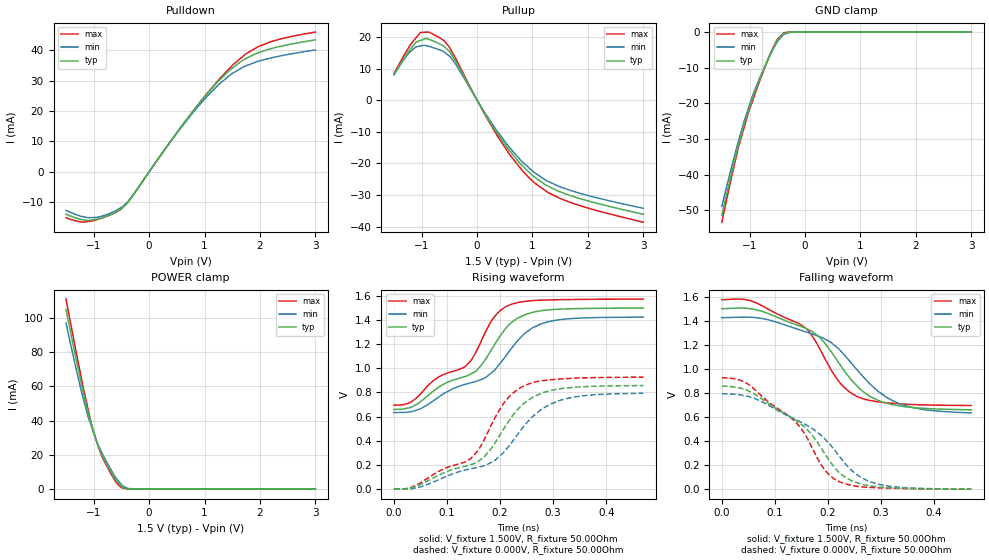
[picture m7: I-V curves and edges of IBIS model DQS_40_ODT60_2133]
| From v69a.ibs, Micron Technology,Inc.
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| MODEL DQS_40_ODT60_2133 (40 Ohm Data Strobe I/O with 60ohm ODT, 1866/2133 Mbps)
[Model]   DQS_40_ODT60_2133
Model_type   I/O
Vinl = 625.000mV
Vinh = 875.000mV
Vmeas = 750.000mV
Vref = 750.000mV
Cref = 0.0pF
Rref = 25.000Ohm
|   typ   min   max
C_comp   1.20pF   1.05pF   1.36pF
| Note: C_comp changes when the ODT circuit is enabled.
[Model Spec]
| Input threshold voltage corners
Vinl   0.6250V   0.5875V   0.6625V
Vinh   0.8750V   0.8375V   0.9125V
| Measurement voltage corners
Vmeas   0.7500V   0.7125V   0.7875V
| Timing spec test load voltage corners
Vref   0.7500V   0.7125V   0.7875V
|[Receiver Thresholds]
|Vth   =  0.750V
|Vth_min  =  0.735V
|Vth_max  =  0.765V
|Vinh_ac  =  0.125V
|Vinh_dc  =  0.100V
|Vinl_ac  = -0.125V
|Vinl_dc  = -0.100V
|Tslew_ac =  5.000ns |Not specified, so set to high value
|Threshold_sensitivity = 0.50
|Reference_supply Pullup_ref
[Receiver Thresholds]
Vcross_low   = 0.625V
Vcross_high  = 0.875V
Vdiff_ac   = 250mV
Vdiff_dc   = 200mV
Tdiffslew_ac = 10.000ns |Not specified, so set to high value
[Voltage Range]   1.5000V   1.4250V   1.5750V
[Pullup Reference]   1.5000V   1.4250V   1.5750V
| Junction Temperature (Ambient temp is 35C typ, 95C min, 0C max)
[Temperature Range]   50.0   110.0   0.0
[Add Submodel]
| Submodel Name   Mode
60ohm_ODT_2133   Non-Driving
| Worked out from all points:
|   slope of the pulldown table from 0 to 0.225 V, typ, clamps not added: 38 ohm
|   slope of the pullup table from 0 to 0.225 V, typ, clamps not added: 33.9 ohm
|   GND clamp passes 1 mA (typ) near -0.42 V on its own axis
|   POWER clamp passes 1 mA (typ) near -0.46 V on its own axis
|   falling waveform, V_fixture 1.500V, R_fixture 50.00Ohm: 20-80 % time 101ps typ, 116ps min, 91.5ps max; typ from 1.5 V to 0.659 V
|   rising waveform, V_fixture 1.500V, R_fixture 50.00Ohm: 20-80 % time 132ps typ, 147ps min, 117ps max; typ from 0.659 V to 1.5 V
|   rising waveform, V_fixture 0.000V, R_fixture 50.00Ohm: 20-80 % time 121ps typ, 135ps min, 108ps max; typ from 0 V to 0.857 V
|   falling waveform, V_fixture 0.000V, R_fixture 50.00Ohm: 20-80 % time 118ps typ, 131ps min, 107ps max; typ from 0.857 V to 0 V
[Pulldown]
|   Voltage   I(typ)   I(min)   I(max)
-1.5V     -13.96mA   -12.69mA   -15.12mA
-1.195V   -15.78mA   -14.77mA   -16.58mA
-955mV    -15.63mA   -15.03mA   -15.81mA
-495mV    -12.08mA   -11.62mA   -12.1mA
-260mV    -6.957mA   -6.872mA   -6.856mA
800mV     20.15mA    19.66mA    20.12mA
1.255V    29.89mA    28.72mA    30.25mA
1.455V    33.47mA    31.73mA    34.11mA
1.74V     37.18mA    34.8mA     38.71mA
1.975V    39.19mA    36.38mA    41.24mA
2.35V     41.19mA    38.05mA    43.59mA
3V        43.39mA    40.08mA    45.95mA
[GND Clamp]
|   Voltage   I(typ)   I(min)   I(max)
-1.5V     -51.33mA   -48.85mA   -53.31mA
-1.32V    -39.2mA    -37.62mA   -40.31mA
-1.2V     -31.7mA    -30.57mA   -32.31mA
-1.1V     -25.85mA   -25.09mA   -26.87mA
-1.02V    -22.1mA    -21.32mA   -22.57mA
-950mV    -18.82mA   -18.03mA   -19.5mA
-850mV    -14.61mA   -14.07mA   -15.14mA
-595mV    -5.207mA   -5.394mA   -4.943mA
-505mV    -2.544mA   -2.91mA    -2.13mA
-380mV    -419.6uA   -621.5uA   -180.2uA
-165mV    0A         -2.918uA   0A
3V        0A         0A         0A
[Pullup]
|   Voltage   I(typ)   I(min)   I(max)
-1.5V     7.95mA     8.248mA    8.388mA
-1.225V   15.63mA    14.98mA    16.85mA
-1.02V    18.85mA    17.12mA    21.4mA
-925mV    19.5mA     17.26mA    21.47mA
-695mV    17.95mA    16.02mA    19.94mA
-505mV    15.48mA    14.01mA    16.93mA
-385mV    12.25mA    11.36mA    13.11mA
360mV     -10.33mA   -9.71mA    -11.13mA
760mV     -19.68mA   -18.43mA   -21mA
1.05V     -24.45mA   -23.07mA   -26.32mA
1.74V     -30.46mA   -28.82mA   -32.66mA
3V        -36.05mA   -34.16mA   -38.55mA
[POWER Clamp]
|   Voltage   I(typ)   I(min)   I(max)
-1.5V     104.9mA    96.95mA    110.8mA
-1.37V    84.07mA    77.64mA    88.84mA
-1.225V   61.86mA    57.37mA    65.04mA
-1.105V   44.83mA    42.59mA    47.13mA
-1.02V    35.67mA    34.63mA    34.86mA
-925mV    25.54mA    26.27mA    25.68mA
-835mV    19.09mA    20.2mA     17.96mA
-600mV    5.255mA    6.588mA    4.139mA
-505mV    1.75mA     2.798mA    931.8uA
-385mV    169.1uA    435.8uA    68.05uA
-260mV    8.657uA    35.03uA    111.5nA
3V        0A         0A         0A
[Ramp]
R_load = 50.00Ohm
|   typ   min   max
dV/dt_r   514.194mV/120.855ps 475.954mV/134.815ps 555.841mV/107.599ps
dV/dt_f   504.129mV/101.355ps 474.729mV/116.386ps 527.439mV/91.470ps
[Falling Waveform]
V_fixture = 1.500V
V_fixture_min = 1.425V
V_fixture_max = 1.575V
R_fixture = 50.00Ohm
|   Time   V(typ)   V(min)   V(max)
0s        1.5V       1.425V     1.574V
55ps      1.498V     1.428V     1.565V
155ps     1.342V     1.312V     1.348V
185ps     1.258V     1.266V     1.162V
220ps     1.053V     1.167V     898mV
255ps     856.3mV    990.5mV    769.5mV
295ps     737.3mV    810.5mV    726.1mV
335ps     691.9mV    709.7mV    709.7mV
385ps     670.6mV    658mV      699.9mV
470ps     659.3mV    633.4mV    695.1mV
[Rising Waveform]
V_fixture = 1.500V
V_fixture_min = 1.425V
V_fixture_max = 1.575V
R_fixture = 50.00Ohm
|   Time   V(typ)   V(min)   V(max)
0s        659.3mV    633.4mV    695.1mV
50ps      723.3mV    664.7mV    787.6mV
85ps      846.4mV    763.4mV    930mV
135ps     933.1mV    868.1mV    1.017V
155ps     977.4mV    891.5mV    1.138V
185ps     1.162V     967.2mV    1.402V
220ps     1.375V     1.157V     1.529V
260ps     1.463V     1.333V     1.561V
295ps     1.486V     1.391V     1.567V
470ps     1.5V       1.425V     1.574V
[Rising Waveform]
V_fixture = 0.000V
V_fixture_min = 0.000V
V_fixture_max = 0.000V
R_fixture = 50.00Ohm
|   Time   V(typ)   V(min)   V(max)
0s        80.86uV    127.7uV    134.6uV
30ps      6.217mV    432.3uV    8.456mV
145ps     201.3mV    167.2mV    253.1mV
160ps     232.3mV    181.1mV    328.8mV
190ps     378.9mV    236.2mV    586.7mV
210ps     520.1mV    320.1mV    729.9mV
240ps     688.2mV    492.9mV    843.6mV
275ps     787.1mV    650.2mV    894.2mV
315ps     831.3mV    737.1mV    912.2mV
470ps     857.1mV    793.4mV    926.5mV
[Falling Waveform]
V_fixture = 0.000V
V_fixture_min = 0.000V
V_fixture_max = 0.000V
R_fixture = 50.00Ohm
|   Time   V(typ)   V(min)   V(max)
0s        857.1mV    793.4mV    926.5mV
45ps      827.1mV    775mV      884.6mV
135ps     585.3mV    586.6mV    574.8mV
155ps     520.4mV    543.7mV    466.8mV
170ps     450.4mV    505.2mV    344.8mV
195ps     287.5mV    413.3mV    154.7mV
220ps     142.4mV    282.3mV    65.42mV
260ps     45.54mV    103.1mV    21.62mV
295ps     19.05mV    40.92mV    11.55mV
470ps     80.86uV    127.7uV    134.6uV
